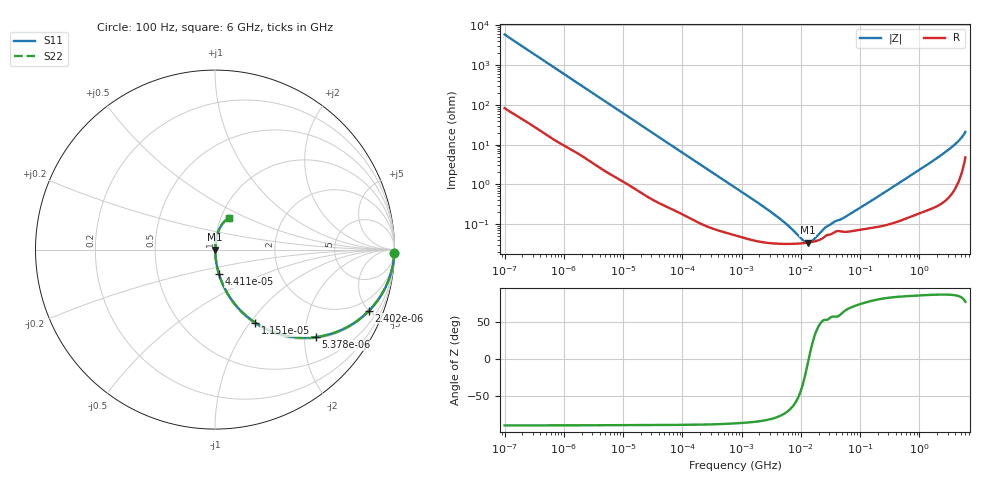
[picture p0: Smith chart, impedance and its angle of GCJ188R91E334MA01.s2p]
!Murata Part Number: GCJ188R91E334MA01
!These Parameters are Measured in Series Mode Connection
!Data Generated on Mar 13, 2026
!  o--ll--o
!Port1  Port2
!  o------o
!Operation Temp=25[degC], DC Bias Voltage=0[V]
!Freq. Start=100[Hz] Stop=6[GHz] 401[Steps]
# Hz S RI R 50
!Freq.(Hz) S11(Real) S11(Imag) S21(Real) S21(Imag) S12(Real) S12(Imag) S22(Real) S22(Imag)
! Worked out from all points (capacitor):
!   401 points, 100 Hz to 6 GHz, reference 50 ohm
!   read as one part in series: C = 272 nF near 109 Hz
!   lowest |Z| = 34.8 mohm at 13.01 MHz (marker M1)
!   series resonance near 13.59 MHz, so ESL is about 510 pH
!   S11 on the Smith chart (normalised r, x): 100 Hz: open; 2.402 kHz: 1.09, -5.02; 5.378 kHz: 1.04, -2.26; 11.51 kHz: 1.02, -1.07; 44.11 kHz: 1.01, -0.28; 6 GHz: 1.10, +0.41
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100  0.9995 -0.0171  0.000534 0.0171  0.000534 0.0171  0.9995 -0.0171
600  0.9884 -0.0996  0.0116 0.0996  0.0116 0.0996  0.9884 -0.0996
2008  0.8956 -0.2972  0.1044 0.2972  0.1044 0.2972  0.8956 -0.2972
2402  0.8587 -0.3397  0.1413 0.3397  0.1413 0.3397  0.8587 -0.3397
5378  0.5601 -0.4876  0.4399 0.4876  0.4399 0.4876  0.5601 -0.4876
7695  0.3883 -0.4782  0.6117 0.4782  0.6117 0.4782  0.3883 -0.4782
11514  0.2256 -0.4083  0.7744 0.4083  0.7744 0.4083  0.2256 -0.4083
19704  0.0941 -0.2821  0.9059 0.2821  0.9059 0.2821  0.0941 -0.2821
40335  0.0264 -0.1497  0.9736 0.1497  0.9736 0.1497  0.0264 -0.1497
44113  0.0226 -0.1376  0.9774 0.1376  0.9774 0.1376  0.0226 -0.1376
135116  0.0036 -0.0467  0.9964 0.0467  0.9964 0.0467  0.0036 -0.0467
774597  0.000598 -0.00838  0.9994 0.00838  0.9994 0.00838  0.000598 -0.00838
3712478  0.000331 -0.00166  0.9997 0.00166  0.9997 0.00166  0.000331 -0.00166
1.087309e7  0.000335 -0.00022  0.9997 0.00022  0.9997 0.00022  0.000335 -0.00022
1.300572e7  0.000345 -4.31e-05  0.9997 4.31e-05  0.9997 4.31e-05  0.000345 -4.31e-05
1.555665e7  0.000361 0.000132  0.9996 -0.000132  0.9996 -0.000132  0.000361 0.000132
2.784235e7  0.00054 0.000706  0.9995 -0.000706  0.9995 -0.000706  0.00054 0.000706
5.449875e7  0.000646 0.00134  0.9994 -0.00134  0.9994 -0.00134  0.000646 0.00134
3.124326e8  0.00106 0.00751  0.9989 -0.00751  0.9989 -0.00751  0.00106 0.00751
2.562649e9  0.00714 0.0595  0.9929 -0.0595  0.9929 -0.0595  0.00714 0.0595
4.193612e9  0.0199 0.105  0.9801 -0.105  0.9801 -0.105  0.0199 0.105
6e9  0.0801 0.1782  0.9199 -0.1782  0.9199 -0.1782  0.0801 0.1782
